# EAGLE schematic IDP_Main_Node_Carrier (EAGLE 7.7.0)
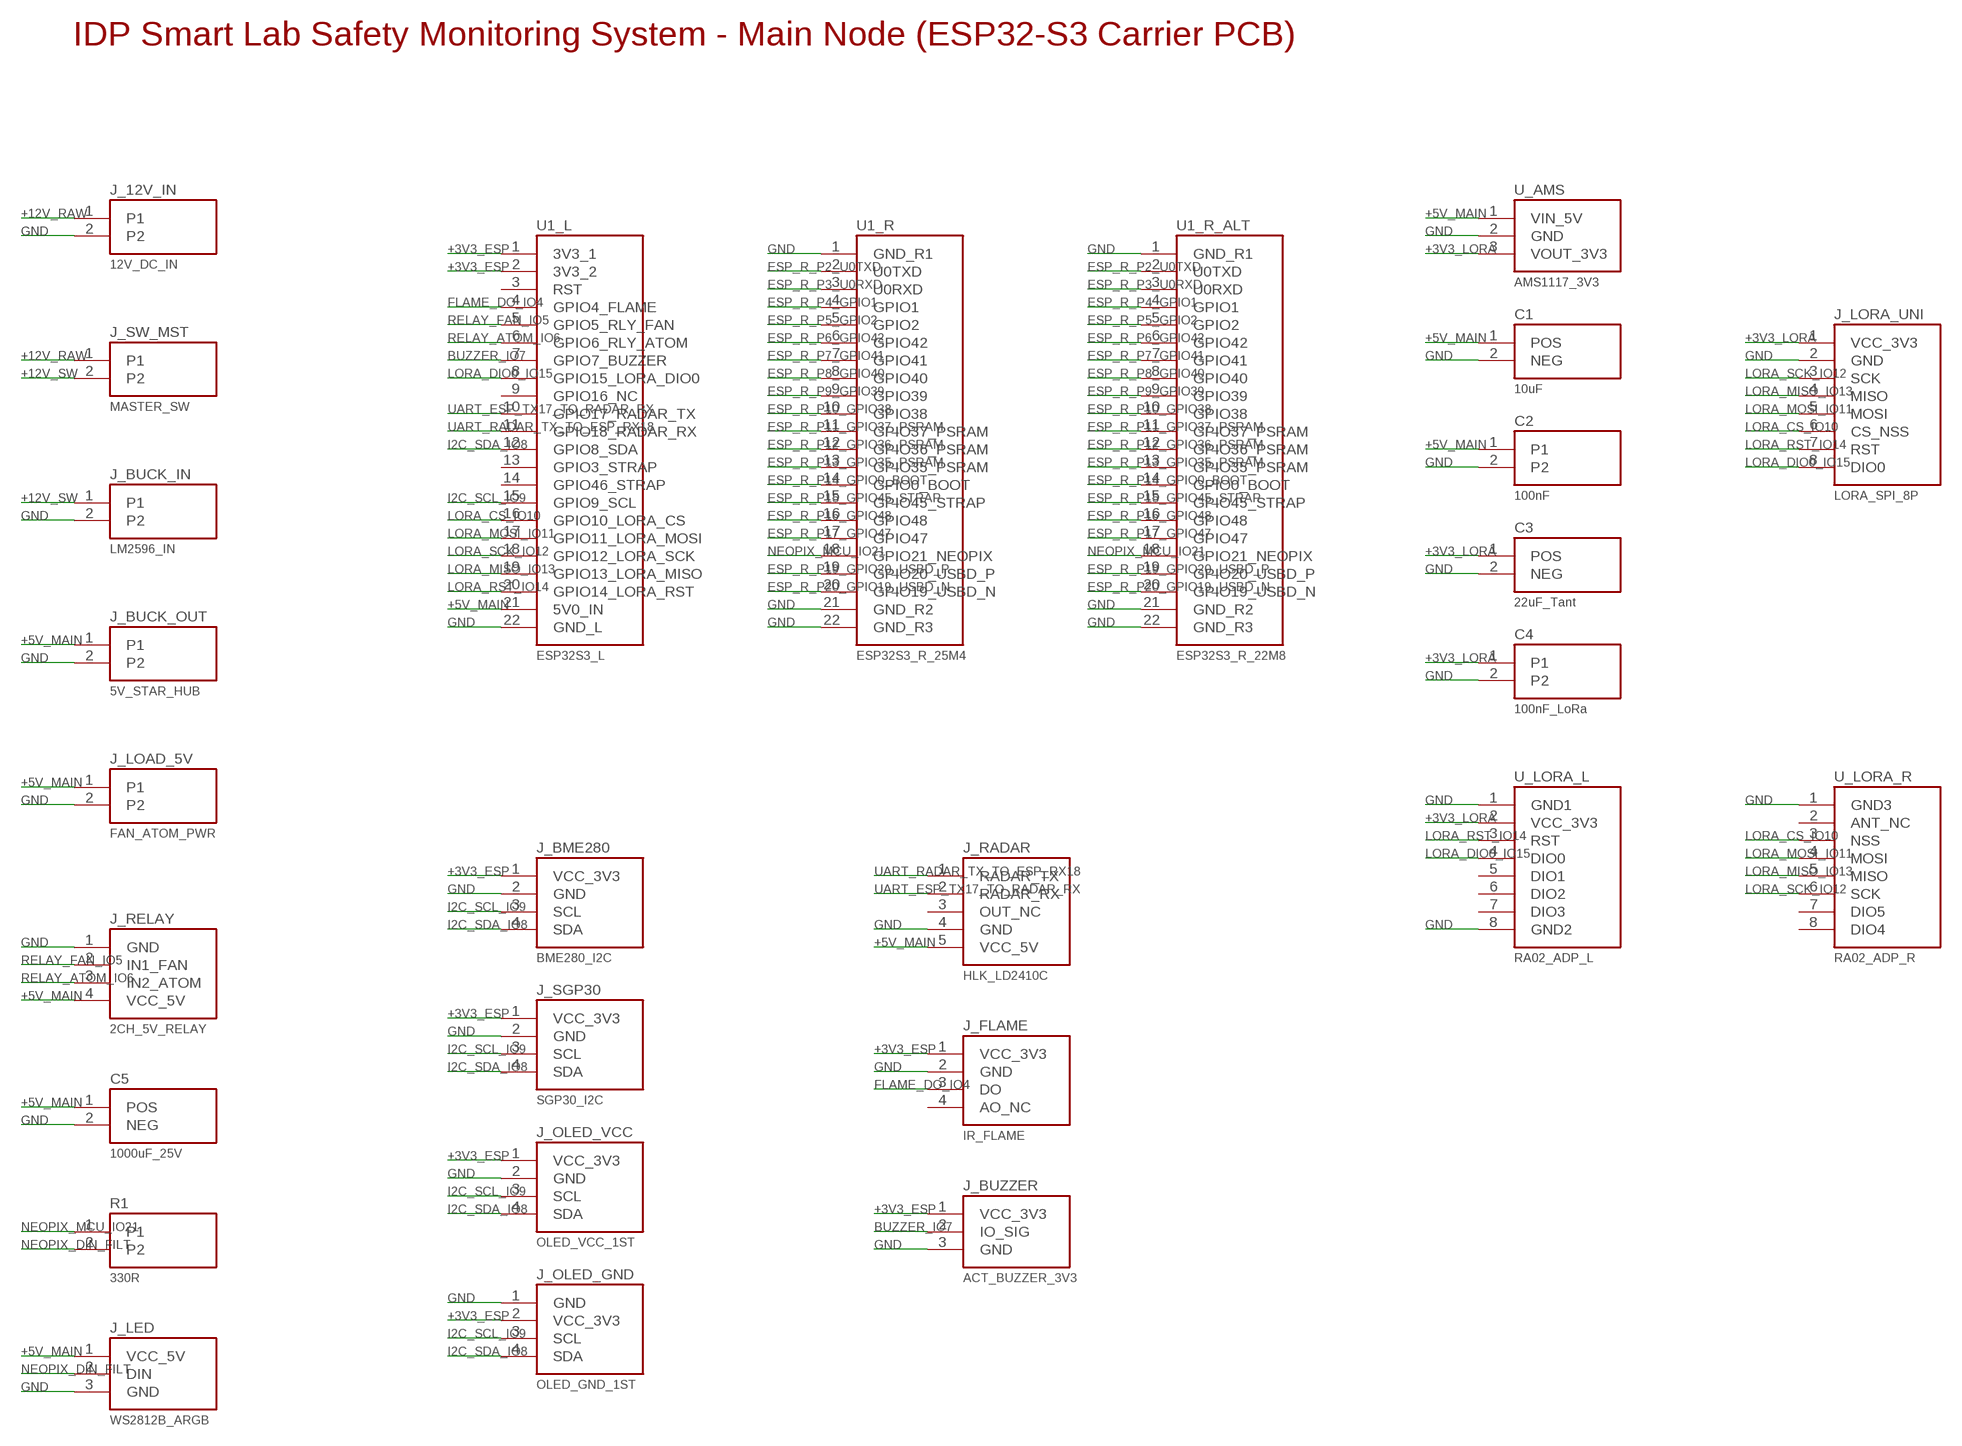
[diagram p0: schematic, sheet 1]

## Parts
C1  10uF  CAP_POL_254  [CAP_RAD_5MM_P254]
C2  100nF  CAP_CER_254  [CAP_DISC_P254]
C3  22uF_Tant  CAP_POL_254  [CAP_RAD_5MM_P254]
C4  100nF_LoRa  CAP_CER_254  [CAP_DISC_P254]
C5  1000uF_25V  CAP_BULK_1000UF  [CAP_ELEC_10MM_P500]
J_12V_IN  12V_DC_IN  KF301_PWR_2P  [KF301_2P_508]
J_BME280  BME280_I2C  I2C_SENSOR_4P  [HDR_1X4]
J_BUCK_IN  LM2596_IN  KF301_PWR_2P  [KF301_2P_508]
J_BUCK_OUT  5V_STAR_HUB  KF301_PWR_2P  [KF301_2P_508]
J_BUZZER  ACT_BUZZER_3V3  BUZZER_3P  [HDR_1X3]
J_FLAME  IR_FLAME  FLAME_SENSOR_4P  [HDR_1X4]
J_LED  WS2812B_ARGB  WS2812B_3P  [HDR_1X3]
J_LOAD_5V  FAN_ATOM_PWR  KF301_PWR_2P  [KF301_2P_508]
J_LORA_UNI  LORA_SPI_8P  LORA_UNI_8P  [HDR_1X8]
J_OLED_GND  OLED_GND_1ST  OLED_GND_FIRST_4P  [HDR_1X4]
J_OLED_VCC  OLED_VCC_1ST  I2C_SENSOR_4P  [HDR_1X4]
J_RADAR  HLK_LD2410C  RADAR_LD2410C_5P  [HDR_1X5]
J_RELAY  2CH_5V_RELAY  RELAY_2CH_4P  [HDR_1X4]
J_SGP30  SGP30_I2C  I2C_SENSOR_4P  [HDR_1X4]
J_SW_MST  MASTER_SW  KF301_PWR_2P  [KF301_2P_508]
R1  330R  RES_330R  [RES_AXIAL_762]
U1_L  ESP32S3_L  ESP32S3_LEFT_22P  [HDR_1X22]
U1_R  ESP32S3_R_25M4  ESP32S3_RIGHT_22P  [HDR_1X22]
U1_R_ALT  ESP32S3_R_22M8  ESP32S3_RIGHT_22P  [HDR_1X22]
U_AMS  AMS1117_3V3  AMS1117_MOD_3P  [HDR_1X3]
U_LORA_L  RA02_ADP_L  LORA_RA02_L8  [HDR_1X8]
U_LORA_R  RA02_ADP_R  LORA_RA02_R8  [HDR_1X8]

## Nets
+3V3_ESP [power]: J_BME280.1(VCC_3V3) J_BUZZER.1(VCC_3V3) J_FLAME.1(VCC_3V3) J_OLED_GND.2(VCC_3V3) J_OLED_VCC.1(VCC_3V3) J_SGP30.1(VCC_3V3) U1_L.1(3V3_1) U1_L.2(3V3_2)
+3V3_LORA [power]: C3.1(POS) C4.1 J_LORA_UNI.1(VCC_3V3) U_AMS.3(VOUT_3V3) U_LORA_L.2(VCC_3V3)
+5V_MAIN [power]: C1.1(POS) C2.1 C5.1(POS) J_BUCK_OUT.1 J_LED.1(VCC_5V) J_LOAD_5V.1 J_RADAR.5(VCC_5V) J_RELAY.4(VCC_5V) U1_L.21(5V0_IN) U_AMS.1(VIN_5V)
+12V_RAW [power]: J_12V_IN.1 J_SW_MST.1
+12V_SW [power]: J_BUCK_IN.1 J_SW_MST.2
BUZZER_IO7: J_BUZZER.2(IO_SIG) U1_L.7(GPIO7_BUZZER)
ESP_R_P2_U0TXD: U1_R.2(U0TXD) U1_R_ALT.2(U0TXD)
ESP_R_P3_U0RXD: U1_R.3(U0RXD) U1_R_ALT.3(U0RXD)
ESP_R_P4_GPIO1: U1_R.4(GPIO1) U1_R_ALT.4(GPIO1)
ESP_R_P5_GPIO2: U1_R.5(GPIO2) U1_R_ALT.5(GPIO2)
ESP_R_P6_GPIO42: U1_R.6(GPIO42) U1_R_ALT.6(GPIO42)
ESP_R_P7_GPIO41: U1_R.7(GPIO41) U1_R_ALT.7(GPIO41)
ESP_R_P8_GPIO40: U1_R.8(GPIO40) U1_R_ALT.8(GPIO40)
ESP_R_P9_GPIO39: U1_R.9(GPIO39) U1_R_ALT.9(GPIO39)
ESP_R_P10_GPIO38: U1_R.10(GPIO38) U1_R_ALT.10(GPIO38)
ESP_R_P11_GPIO37_PSRAM: U1_R.11(GPIO37_PSRAM) U1_R_ALT.11(GPIO37_PSRAM)
ESP_R_P12_GPIO36_PSRAM: U1_R.12(GPIO36_PSRAM) U1_R_ALT.12(GPIO36_PSRAM)
ESP_R_P13_GPIO35_PSRAM: U1_R.13(GPIO35_PSRAM) U1_R_ALT.13(GPIO35_PSRAM)
ESP_R_P14_GPIO0_BOOT: U1_R.14(GPIO0_BOOT) U1_R_ALT.14(GPIO0_BOOT)
ESP_R_P15_GPIO45_STRAP: U1_R.15(GPIO45_STRAP) U1_R_ALT.15(GPIO45_STRAP)
ESP_R_P16_GPIO48: U1_R.16(GPIO48) U1_R_ALT.16(GPIO48)
ESP_R_P17_GPIO47: U1_R.17(GPIO47) U1_R_ALT.17(GPIO47)
ESP_R_P19_GPIO20_USBD_P: U1_R.19(GPIO20_USBD_P) U1_R_ALT.19(GPIO20_USBD_P)
ESP_R_P20_GPIO19_USBD_N: U1_R.20(GPIO19_USBD_N) U1_R_ALT.20(GPIO19_USBD_N)
FLAME_DO_IO4: J_FLAME.3(DO) U1_L.4(GPIO4_FLAME)
GND [power]: C1.2(NEG) C2.2 C3.2(NEG) C4.2 C5.2(NEG) J_12V_IN.2 J_BME280.2(GND) J_BUCK_IN.2 J_BUCK_OUT.2 J_BUZZER.3(GND) J_FLAME.2(GND) J_LED.3(GND) J_LOAD_5V.2 J_LORA_UNI.2(GND) J_OLED_GND.1(GND) J_OLED_VCC.2(GND) J_RADAR.4(GND) J_RELAY.1(GND) J_SGP30.2(GND) U1_L.22(GND_L) U1_R.1(GND_R1) U1_R.21(GND_R2) U1_R.22(GND_R3) U1_R_ALT.1(GND_R1) U1_R_ALT.21(GND_R2) U1_R_ALT.22(GND_R3) U_AMS.2(GND) U_LORA_L.1(GND1) U_LORA_L.8(GND2) U_LORA_R.1(GND3)
I2C_SCL_IO9: J_BME280.3(SCL) J_OLED_GND.3(SCL) J_OLED_VCC.3(SCL) J_SGP30.3(SCL) U1_L.15(GPIO9_SCL)
I2C_SDA_IO8: J_BME280.4(SDA) J_OLED_GND.4(SDA) J_OLED_VCC.4(SDA) J_SGP30.4(SDA) U1_L.12(GPIO8_SDA)
LORA_CS_IO10: J_LORA_UNI.6(CS_NSS) U1_L.16(GPIO10_LORA_CS) U_LORA_R.3(NSS)
LORA_DIO0_IO15: J_LORA_UNI.8(DIO0) U1_L.8(GPIO15_LORA_DIO0) U_LORA_L.4(DIO0)
LORA_MISO_IO13: J_LORA_UNI.4(MISO) U1_L.19(GPIO13_LORA_MISO) U_LORA_R.5(MISO)
LORA_MOSI_IO11: J_LORA_UNI.5(MOSI) U1_L.17(GPIO11_LORA_MOSI) U_LORA_R.4(MOSI)
LORA_RST_IO14: J_LORA_UNI.7(RST) U1_L.20(GPIO14_LORA_RST) U_LORA_L.3(RST)
LORA_SCK_IO12: J_LORA_UNI.3(SCK) U1_L.18(GPIO12_LORA_SCK) U_LORA_R.6(SCK)
NEOPIX_DIN_FILT: J_LED.2(DIN) R1.2
NEOPIX_MCU_IO21: R1.1 U1_R.18(GPIO21_NEOPIX) U1_R_ALT.18(GPIO21_NEOPIX)
RELAY_ATOM_IO6: J_RELAY.3(IN2_ATOM) U1_L.6(GPIO6_RLY_ATOM)
RELAY_FAN_IO5: J_RELAY.2(IN1_FAN) U1_L.5(GPIO5_RLY_FAN)
UART_ESP_TX17_TO_RADAR_RX: J_RADAR.2(RADAR_RX) U1_L.10(GPIO17_RADAR_TX)
UART_RADAR_TX_TO_ESP_RX18: J_RADAR.1(RADAR_TX) U1_L.11(GPIO18_RADAR_RX)
Unconnected: J_FLAME.4(AO_NC) J_RADAR.3(OUT_NC) U1_L.3(RST) U1_L.9(GPIO16_NC) U1_L.13(GPIO3_STRAP) U1_L.14(GPIO46_STRAP) U_LORA_L.5(DIO1) U_LORA_L.6(DIO2) U_LORA_L.7(DIO3) U_LORA_R.2(ANT_NC) U_LORA_R.7(DIO5) U_LORA_R.8(DIO4)

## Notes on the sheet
- IDP Smart Lab Safety Monitoring System - Main Node (ESP32-S3 Carrier PCB)

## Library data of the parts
C1 C3 = IDP_Lab_Safety:CAP_POL_254
C2 C4 = IDP_Lab_Safety:CAP_CER_254
C5 = IDP_Lab_Safety:CAP_BULK_1000UF
J_12V_IN J_BUCK_IN J_BUCK_OUT J_LOAD_5V J_SW_MST = IDP_Lab_Safety:KF301_PWR_2P
J_BME280 J_OLED_VCC J_SGP30 = IDP_Lab_Safety:I2C_SENSOR_4P
J_BUZZER = IDP_Lab_Safety:BUZZER_3P
J_FLAME = IDP_Lab_Safety:FLAME_SENSOR_4P
J_LED = IDP_Lab_Safety:WS2812B_3P
J_LORA_UNI = IDP_Lab_Safety:LORA_UNI_8P
J_OLED_GND = IDP_Lab_Safety:OLED_GND_FIRST_4P
J_RADAR = IDP_Lab_Safety:RADAR_LD2410C_5P
J_RELAY = IDP_Lab_Safety:RELAY_2CH_4P
R1 = IDP_Lab_Safety:RES_330R
U1_L = IDP_Lab_Safety:ESP32S3_LEFT_22P
U1_R U1_R_ALT = IDP_Lab_Safety:ESP32S3_RIGHT_22P
U_AMS = IDP_Lab_Safety:AMS1117_MOD_3P
U_LORA_L = IDP_Lab_Safety:LORA_RA02_L8
U_LORA_R = IDP_Lab_Safety:LORA_RA02_R8

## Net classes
0 default: width 0.3 mm
1 power: width 0.8 mm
